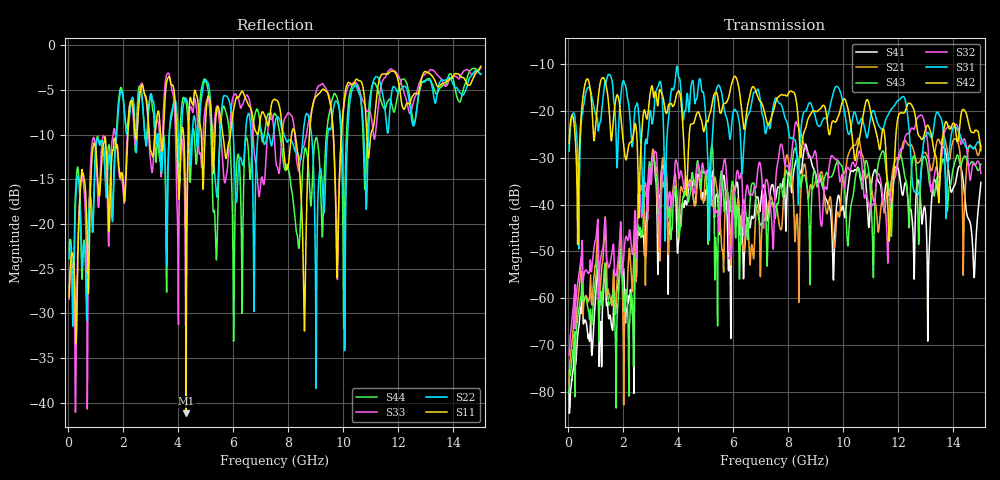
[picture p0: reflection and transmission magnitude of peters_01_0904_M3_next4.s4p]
# MHZ S RI R 50.00
! FREQ  S11  S12  S13  S14
!  S21  S22  S23  S24
!  S31  S32  S33  S34
!  S41  S42  S43  S44
!  REAL  IMAG  REAL  IMAG  REAL  IMAG  REAL  IMAG
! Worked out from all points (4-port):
!   1496 points, 50 MHz to 15 GHz, reference 50 ohm
!   strongest paths, dB at 50 MHz, 3.79 GHz, 7.53 GHz, 11.27 GHz, 15 GHz:
!     S42: -27.0, -18.8, -18.6, -26.5, -28.5
!     S31: -28.6, -15.2, -17.4, -22.9, -27.8
!     S32: -72.2, -38.8, -37.3, -33.4, -33.3
!     S43: -80.3, -45.3, -43.0, -31.4, -31.4
!     S21: -78.5, -38.3, -40.5, -45.8, -27.5
!     S41: -79.8, -38.9, -38.8, -34.9, -35.3
!   lowest |S11| = -41.2 dB at 4.3 GHz (marker M1), VSWR 1.02, Z = 49.5 + j0.694 ohm
!   |S11| at or under -10 dB: start of sweep to 2.18 GHz; 7.803 GHz to 8.123 GHz (320.3 MHz wide, 4.02 % of centre); 8.261 GHz to 8.775 GHz (513.5 MHz wide, 6.03 % of centre)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
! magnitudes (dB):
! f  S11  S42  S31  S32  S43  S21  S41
! 50 MHz  -28.1  -27.0  -28.6  -72.2  -80.3  -78.5  -79.8
! 2.36 GHz  -6.6  -25.9  -27.0  -50.4  -62.7  -57.5  -64.0
! 3.06 GHz  -12.2  -14.6  -22.7  -33.1  -31.0  -31.2  -30.4
! 4.3 GHz  -41.2  -38.0  -18.5  -34.2  -36.4  -35.0  -39.9
! 6.07 GHz  -6.4  -12.6  -19.7  -37.0  -42.8  -38.4  -36.8
! 11.69 GHz  -3.0  -46.6  -20.2  -40.1  -38.5  -37.5  -38.0
! 15 GHz  -2.3  -28.5  -27.8  -33.3  -31.4  -27.5  -35.3
